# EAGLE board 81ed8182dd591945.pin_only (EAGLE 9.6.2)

Size 71.75 x 54.61 mm. Coordinates in mm from the lower left corner, seen from the top.
Copper layers (1*16): Top 0.035mm / dielectric 1.5mm / Bottom 0.035mm
Design rules "SparkFun10mil": minimum track width 10mil, minimum drill 20mil, track to track 10mil, track to pad 10mil, pad to pad 10mil, via to via 10mil, smd to smd 10mil, copper to edge 10mil, drill to drill 10mil, minimum pad ring 12mil, minimum via ring 10mil, stop-mask expansion 4mil, vias tented up to drill 25mil, thermal gap 10mil

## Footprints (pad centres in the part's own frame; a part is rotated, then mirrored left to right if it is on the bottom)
1X23_ROUND_70MIL = drill 1 pad 1.676: 1 -27.94,0; 2 -25.4,0; 3 -22.86,0; 4 -20.32,0; 5 -17.78,0; 6 -15.24,0; 7 -12.7,0; 8 -10.16,0; 9 -7.62,0; 10 -5.08,0; 11 -2.54,0; 12 0,0; 13 2.54,0; 14 5.08,0; 15 7.62,0; 16 10.16,0; 17 12.7,0; 18 15.24,0; 19 17.78,0; 20 20.32,0; 21 22.86,0; 22 25.4,0; 23 27.94,0
1X11_ROUND_76 = drill 1 pad 1.93: 1 -12.7,0; 2 -10.16,0; 3 -7.62,0; 4 -5.08,0; 5 -2.54,0; 6 0,0; 7 2.54,0; 8 5.08,0; 9 7.62,0; 10 10.16,0; 11 12.7,0
1X08_ROUND_70 = drill 1 pad 1.778: 1 -8.89,0; 2 -6.35,0; 3 -3.81,0; 4 -1.27,0; 5 1.27,0; 6 3.81,0; 7 6.35,0; 8 8.89,0
1X04_ROUND_76 = drill 1 pad 1.93: 1 -3.81,0; 2 -1.27,0; 3 1.27,0; 4 3.81,0
1X06_ROUND_76 = drill 1 pad 1.93: 1 -6.35,0; 2 -3.81,0; 3 -1.27,0; 4 1.27,0; 5 3.81,0; 6 6.35,0
1X03_ROUND_76 = drill 1 pad 1.93: 1 -2.54,0; 2 0,0; 3 2.54,0
BREAKOUT_SOIC8 = smd 0.66 x 3.81: 1 -1.905,-4.14; 2 -0.635,-4.14; 3 0.635,-4.14; 4 1.905,-4.14; 5 1.905,4.14; 6 0.635,4.14; 7 -0.635,4.14; 8 -1.905,4.14
BREAKOUT_SOT23-6 = smd 0.55 x 1.6: 1 -0.95,-1.5; 2 0,-1.5; 3 0.95,-1.5; 4 0.95,1.5; 5 0,1.5; 6 -0.95,1.5
BEAGLEBONE_SHIELD = drill 1 square: 1 4.445,19.05; 47 52.705,19.05 | drill 1: 2 1.905,19.05; 3 4.445,21.59; 4 1.905,21.59; 5 4.445,24.13; 6 1.905,24.13; 7 4.445,26.67; 8 1.905,26.67; 9 4.445,29.21; 10 1.905,29.21; 11 4.445,31.75; 12 1.905,31.75; 13 4.445,34.29; 14 1.905,34.29; 15 4.445,36.83; 16 1.905,36.83; 17 4.445,39.37; 18 1.905,39.37; 19 4.445,41.91; 20 1.905,41.91; 21 4.445,44.45; 22 1.905,44.45; 23 4.445,46.99; 24 1.905,46.99; 25 4.445,49.53; 26 1.905,49.53; 27 4.445,52.07; 28 1.905,52.07; 29 4.445,54.61; 30 1.905,54.61; 31 4.445,57.15; 32 1.905,57.15; 33 4.445,59.69; 34 1.905,59.69; 35 4.445,62.23; 36 1.905,62.23; 37 4.445,64.77; 38 1.905,64.77; 39 4.445,67.31; 40 1.905,67.31; 41 4.445,69.85; 42 1.905,69.85; 43 4.445,72.39; 44 1.905,72.39; 45 4.445,74.93; 46 1.905,74.93; 48 50.165,19.05; 49 52.705,21.59; 50 50.165,21.59; 51 52.705,24.13; 52 50.165,24.13; 53 52.705,26.67; 54 50.165,26.67; 55 52.705,29.21; 56 50.165,29.21; 57 52.705,31.75; 58 50.165,31.75; 59 52.705,34.29; 60 50.165,34.29; 61 52.705,36.83; 62 50.165,36.83; 63 52.705,39.37; 64 50.165,39.37; 65 52.705,41.91; 66 50.165,41.91; 67 52.705,44.45; 68 50.165,44.45; 69 52.705,46.99; 70 50.165,46.99; 71 52.705,49.53; 72 50.165,49.53; 73 52.705,52.07; 74 50.165,52.07; 75 52.705,54.61; 76 50.165,54.61; 77 52.705,57.15; 78 50.165,57.15; 79 52.705,59.69; 80 50.165,59.69; 81 52.705,62.23; 82 50.165,62.23; 83 52.705,64.77; 84 50.165,64.77; 85 52.705,67.31; 86 50.165,67.31; 87 52.705,69.85; 88 50.165,69.85; 89 52.705,72.39; 90 50.165,72.39; 91 52.705,74.93; 92 50.165,74.93
MOUNTINGHOLE_3.0_PLATEDTHIN = drill 3 pad 3.6: P$1 0,0

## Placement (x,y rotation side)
JP1  [1X23_ROUND_70MIL]  32.39,45.09 180 top
JP2  [1X23_ROUND_70MIL]  32.39,47.62 0 top
JP3  [1X23_ROUND_70MIL]  32.39,6.99 180 top
JP4  [1X23_ROUND_70MIL]  32.39,9.53 0 top
JP5  [1X11_ROUND_76]  42.55,27.3 90 top
JP6  [1X11_ROUND_76]  45.08,27.3 90 top
JP7  V_3.3V  [1X08_ROUND_70]  56.52,34.92 0 top
JP8  V_GND  [1X08_ROUND_70]  56.52,32.38 0 top
JP9  [1X04_ROUND_76]  65.41,20.95 270 top
JP10  [1X04_ROUND_76]  67.94,20.95 90 top
JP11  [1X11_ROUND_76]  9.52,27.3 90 top
JP12  [1X11_ROUND_76]  12.07,27.3 90 top
JP13  [1X11_ROUND_76]  14.61,27.3 90 top
JP14  [1X11_ROUND_76]  17.14,27.3 90 top
JP15  [1X11_ROUND_76]  19.68,27.3 90 top
JP16  [1X11_ROUND_76]  22.22,27.3 90 top
JP17  [1X11_ROUND_76]  24.76,27.3 90 top
JP18  [1X11_ROUND_76]  27.3,27.3 90 top
JP19  [1X11_ROUND_76]  29.85,27.3 90 top
JP20  [1X11_ROUND_76]  32.39,27.3 90 top
JP21  [1X11_ROUND_76]  34.92,27.3 90 top
JP22  [1X11_ROUND_76]  37.47,27.3 90 top
JP23  [1X11_ROUND_76]  40,27.3 90 top
JP24  V_5V  [1X08_ROUND_70]  56.52,37.47 0 top
JP26  [1X06_ROUND_76]  47.62,20.95 90 top
JP34  [1X03_ROUND_76]  52.7,24.77 90 top
JP35  [1X03_ROUND_76]  52.7,17.14 90 top
U1  [BREAKOUT_SOIC8]  60.58,21.59 0 top
U2  [BREAKOUT_SOT23-6]  55.88,20.95 180 top
U$2  BEAGLEBONE_OUTLINE  [BEAGLEBONE_SHIELD]  -14.61,54.61 270 top
U$7  [ADAFRUIT200MIL]  66.8,43.05 270 top
U$22  MOUNTINGHOLE3.0THIN  [MOUNTINGHOLE_3.0_PLATEDTHIN]  65.44,48.3 0 top
U$23  MOUNTINGHOLE3.0THIN  [MOUNTINGHOLE_3.0_PLATEDTHIN]  65.44,6.32 0 top

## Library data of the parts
JP1-JP24 JP26 JP34 JP35 U1 U2 U$2 U$22 U$23 = microbuilder
U$7 = adafruit

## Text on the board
tPlace: 2 | P8 | 1 | 9 | 1 | 3 | 5 | 7 | 11 | 13 | 15 | 17 | 19 | 21 | 23 | 25 | 27 | 29 | 31 | 33 | 35 | 37 | 39 | 41 | 43 | 45 | adafruit! | 5.0V | 3.3V | GND | 1 | 4 | 5 | SOIC8 | Beagle Bone Proto | SOT23-6 | 6 | 1 | 8 | 2 | 4\ | 6 | 8 | 10 | 12 | 14 | 16 | 18 | 20 | 22 | 24 | 26 | 28 | 30 | 32 | 34 | 36 | 38 | 40 | 42 | 44 | 46 | 2 | P9 | 1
